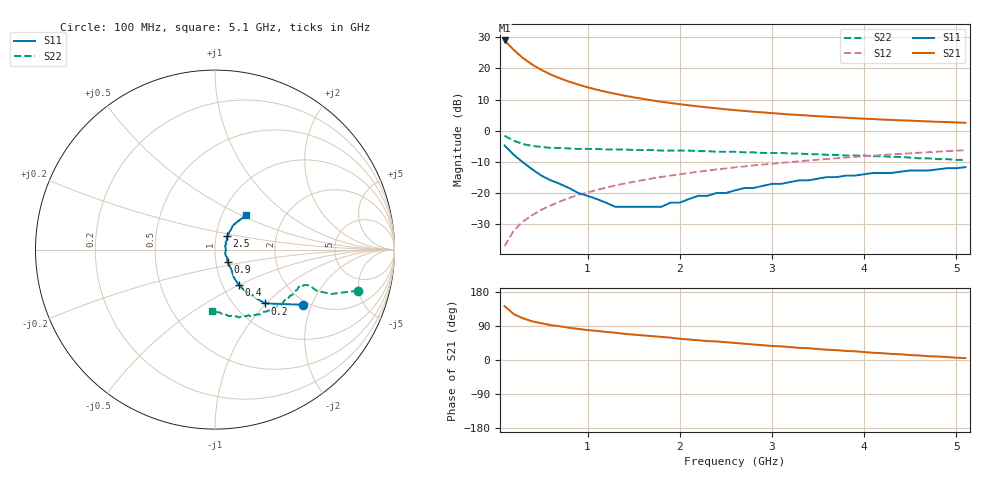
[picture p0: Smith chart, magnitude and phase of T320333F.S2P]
!AT-32033
!S PARAMETERS at Vce=2.7V  Ic=15mA.  LAST UPDATED 01-05-95
# ghz s ma r 50
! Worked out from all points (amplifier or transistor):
!   51 points, 100 MHz to 5.1 GHz, reference 50 ohm
!   highest |S21| = 29.0 dB at 100 MHz (marker M1)
!   |S21| within 3 dB of that: start of sweep to 198 MHz
!   unconditionally stable (mu >= 1): 796.1 MHz to 2.067 GHz; 2.126 GHz to 2.257 GHz; 2.394915 GHz to 2.404102 GHz
!   at 900 MHz: K = 1.01, MAG = 17.2 dB, |S12| = -20.6 dB
!   at 2.6 GHz: K = 0.99, MSG = 9.2 dB, |S12| = -11.8 dB
!   at 5.1 GHz: K = 0.94, MSG = 4.4 dB, |S12| = -6.2 dB
!   S11 on the Smith chart (normalised r, x): 100 MHz: 1.88, -1.74; 200 MHz: 1.37, -0.98; 400 MHz: 1.19, -0.50; 900 MHz: 1.14, -0.16; 2.5 GHz: 1.13, +0.17; 5.1 GHz: 1.30, +0.54
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0.1  0.58 -32.0  28.17 142.0  0.014 77.0  0.83 -16.0
0.2  0.41 -47.0  19.8 121.0  0.025 74.0  0.69 -21.0
0.3  0.31 -53.0  14.67 110.0  0.035 75.0  0.61 -22.0
0.4  0.24 -56.0  11.53 102.0  0.044 75.0  0.57 -21.0
0.5  0.19 -56.0  9.47 97.0  0.054 75.0  0.55 -21.0
0.6  0.16 -53.0  8.01 92.0  0.063 75.0  0.53 -22.0
0.7  0.14 -50.0  6.95 89.0  0.073 75.0  0.53 -23.0
0.8  0.12 -48.0  6.14 85.0  0.083 74.0  0.52 -23.0
0.9  0.1 -45.0  5.51 82.0  0.093 73.0  0.51 -24.0
1  0.09 -41.0  4.99 79.0  0.102 73.0  0.51 -25.0
1.2  0.07 -30.0  4.21 74.0  0.122 71.0  0.5 -28.0
1.3  0.06 -20.0  3.92 72.0  0.132 70.0  0.5 -29.0
1.4  0.06 -11.0  3.66 69.0  0.142 69.0  0.5 -30.0
1.6  0.06 4.0  3.25 65.0  0.161 67.0  0.49 -33.0
1.8  0.06 21.0  2.92 61.0  0.181 65.0  0.48 -35.0
2.1  0.08 37.0  2.56 54.0  0.21 62.0  0.48 -40.0
2.5  0.1 48.0  2.21 47.0  0.248 58.0  0.46 -46.0
2.6  0.11 48.0  2.14 45.0  0.258 57.0  0.46 -47.0
3  0.14 51.0  1.92 37.0  0.295 52.0  0.44 -53.0
3.5  0.17 53.0  1.71 29.0  0.343 47.0  0.42 -62.0
4.3  0.21 50.0  1.49 16.0  0.416 38.0  0.38 -76.0
5.1  0.26 48.0  1.34 5.0  0.487 28.0  0.34 -93.0
